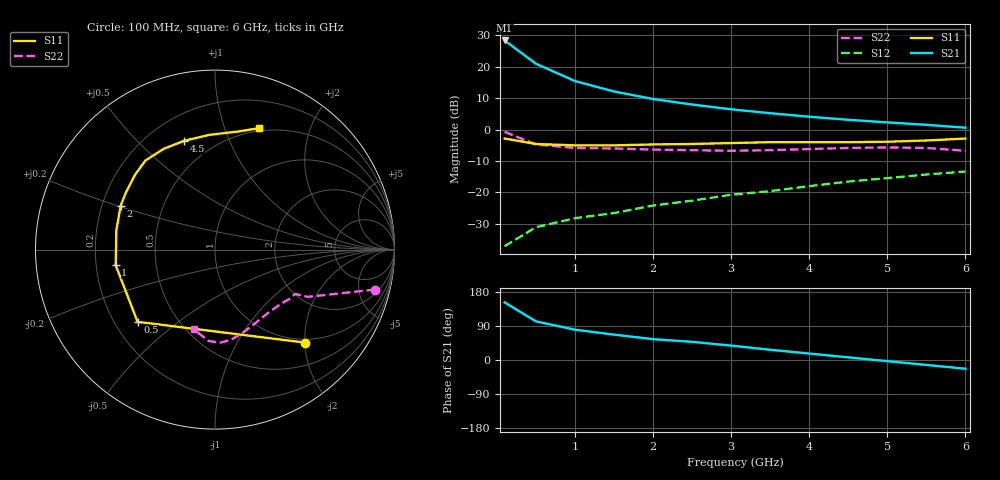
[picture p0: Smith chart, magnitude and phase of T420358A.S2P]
!AT-42035
!S AND NOISE PARAMETERS at Vce=8V  Ic=10mA.  LAST UPDATED 07-21-92
# ghz s ma r 50
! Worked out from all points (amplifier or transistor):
!   13 points, 100 MHz to 6 GHz, reference 50 ohm
!   highest |S21| = 28.3 dB at 100 MHz (marker M1)
!   |S21| within 3 dB of that: start of sweep to 262.2 MHz
!   unconditionally stable (mu >= 1): 1.061 GHz to 3.812 GHz
!   at 1 GHz: K = 0.98, MSG = 21.8 dB, |S12| = -28.2 dB
!   at 3 GHz: K = 1.11, MAG = 11.6 dB, |S12| = -20.7 dB
!   at 6 GHz: K = 0.71, MSG = 7.0 dB, |S12| = -13.4 dB
!   lowest NFmin = 1.00 dB at 100 MHz
!   S11 on the Smith chart (normalised r, x): 100 MHz: 0.93, -2.00; 500 MHz: 0.29, -0.36; 1 GHz: 0.28, -0.07; 2 GHz: 0.28, +0.21; 4.5 GHz: 0.35, +0.69; 6 GHz: 0.47, +1.32
0.1  0.72 -46.0  26.09 152.0  0.014 73.0  0.92 -14.0
0.5  0.59 -137.0  11.13 102.0  0.028 44.0  0.58 -27.0
1  0.56 -171.0  5.91 80.0  0.039 47.0  0.51 -29.0
1.5  0.56 169.0  4.03 67.0  0.047 52.0  0.5 -33.0
2  0.58 155.0  3.06 55.0  0.062 55.0  0.48 -38.0
2.5  0.59 147.0  2.5 48.0  0.074 61.0  0.47 -42.0
3  0.61 137.0  2.1 38.0  0.092 65.0  0.46 -51.0
3.5  0.63 128.0  1.82 27.0  0.105 62.0  0.47 -63.0
4  0.63 117.0  1.6 17.0  0.126 57.0  0.49 -72.0
4.5  0.63 106.0  1.43 7.0  0.149 53.0  0.51 -80.0
5  0.64 93.0  1.3 -3.0  0.169 48.0  0.52 -87.0
5.5  0.67 79.0  1.19 -13.0  0.193 41.0  0.51 -94.0
6  0.72 70.0  1.07 -23.0  0.215 35.0  0.46 -105.0
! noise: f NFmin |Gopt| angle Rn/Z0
0.1  1  0.04  10  0.13
0.5  1.1  0.04  66  0.12
1  1.3  0.07  150  0.12
2  2  0.2  -178  0.12
4  3  0.51  -110  0.36
